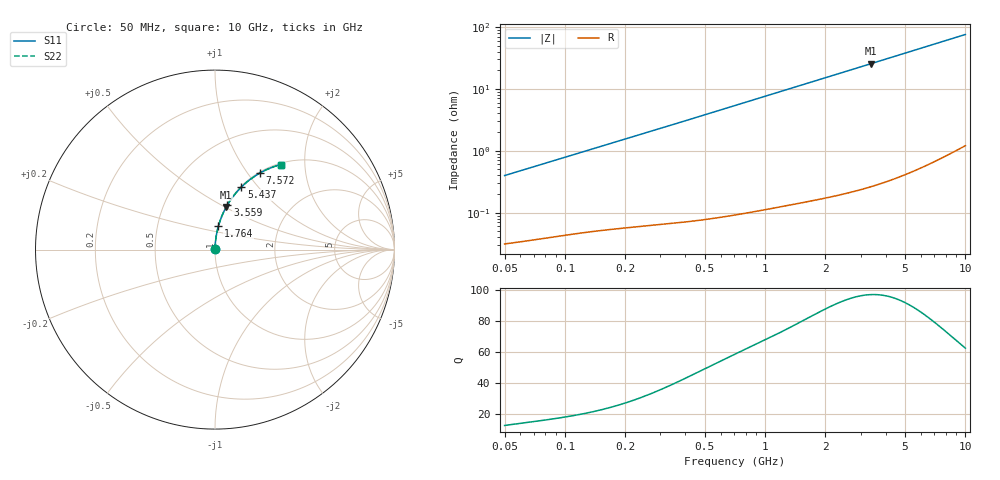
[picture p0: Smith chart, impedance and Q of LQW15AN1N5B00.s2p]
!Murata Part Number: LQW15AN1N5B00
!These Parameters are Measured in Series Mode Connection
!  o--[Z]--o
!Port1  Port2
!  o-------o
!Freq. Start=50[MHz] Stop=10[GHz], 401[Steps]
# Hz S RI R 50
!Freq.(Hz)	S 11(Real)	S 11(Imag)	S 21(Real)	S 21(Imag)	S 12(Real)	S 12(Imag)	S 22(Real)	S 22(Imag)
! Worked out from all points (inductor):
!   401 points, 50 MHz to 10 GHz, reference 50 ohm
!   read as one part in series: L = 1.26 nH near 51.34 MHz
!   highest Q = 97.1 at 3.375 GHz (marker M1), where L = 1.2 nH
!   S11 on the Smith chart (normalised r, x): 50 MHz: 1.00, +0.01; 1.764 GHz: 1.00, +0.27; 3.559 GHz: 1.01, +0.54; 5.437 GHz: 1.01, +0.82; 7.572 GHz: 1.02, +1.14; 10 GHz: 1.02, +1.51
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5e7  0.000328 0.00396  0.9997 -0.00396  0.9997 -0.00396  0.000328 0.00396
5.134228e7  0.000333 0.00407  0.9997 -0.00407  0.9997 -0.00407  0.000333 0.00407
1.214486e8  0.00056 0.00943  0.9994 -0.00943  0.9994 -0.00943  0.00056 0.00943
2.949953e8  0.00115 0.0225  0.9989 -0.0225  0.9989 -0.0225  0.00115 0.0225
4.689809e8  0.00203 0.0357  0.998 -0.0357  0.998 -0.0357  0.00203 0.0357
7.071068e8  0.00379 0.0535  0.9962 -0.0535  0.9962 -0.0535  0.00379 0.0535
1.139142e9  0.00859 0.0855  0.9914 -0.0855  0.9914 -0.0855  0.00859 0.0855
1.408053e9  0.0126 0.1052  0.9874 -0.1052  0.9874 -0.1052  0.0126 0.1052
1.717543e9  0.0181 0.1274  0.9819 -0.1274  0.9819 -0.1274  0.0181 0.1274
1.763651e9  0.019 0.1307  0.981 -0.1307  0.981 -0.1307  0.019 0.1307
2.455993e9  0.0351 0.1787  0.9649 -0.1787  0.9649 -0.1787  0.0351 0.1787
2.917498e9  0.0483 0.2092  0.9517 -0.2092  0.9517 -0.2092  0.0483 0.2092
3.375117e9  0.0631 0.2381  0.9369 -0.2381  0.9369 -0.2381  0.0631 0.2381
3.558764e9  0.0695 0.2493  0.9305 -0.2493  0.9305 -0.2493  0.0695 0.2493
4.171863e9  0.0927 0.2848  0.9073 -0.2848  0.9073 -0.2848  0.0927 0.2848
4.762728e9  0.1171 0.3162  0.8829 -0.3162  0.8829 -0.3162  0.1171 0.3162
5.437278e9  0.1469 0.3485  0.8531 -0.3485  0.8531 -0.3485  0.1469 0.3485
6.458996e9  0.195 0.3902  0.805 -0.3902  0.805 -0.3902  0.195 0.3902
7.571744e9  0.2492 0.426  0.7508 -0.426  0.7508 -0.426  0.2492 0.426
8.876195e9  0.3127 0.4563  0.6873 -0.4563  0.6873 -0.4563  0.3127 0.4563
9.738562e9  0.3535 0.4703  0.6465 -0.4703  0.6465 -0.4703  0.3535 0.4703
1e10  0.3656 0.4737  0.6344 -0.4737  0.6344 -0.4737  0.3656 0.4737
